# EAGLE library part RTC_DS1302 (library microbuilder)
DS1302 Trickle-Charge Timekeeping Chip
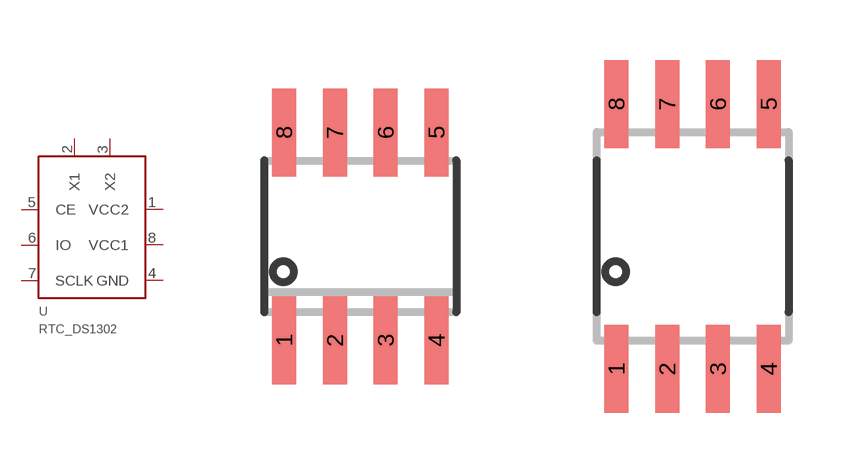
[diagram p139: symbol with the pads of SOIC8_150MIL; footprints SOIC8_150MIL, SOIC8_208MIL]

Designator prefix U

## RTC_DS1302150  [SOIC8_150MIL]
1  VCC2
2  X1
3  X2
4  GND
5  CE
6  IO
7  SCLK
8  VCC1

## RTC_DS1302208  [SOIC8_208MIL]
Pads as for SOIC8_150MIL

## Footprint SOIC8_150MIL (pad centres in mm)
Small Outline IC - 150mil Wide
smd 0.6 x 2.2: 1 -1.905,-2.6; 2 -0.635,-2.6; 3 0.635,-2.6; 4 1.905,-2.6; 5 1.905,2.6; 6 0.635,2.6; 7 -0.635,2.6; 8 -1.905,2.6

## Footprint SOIC8_208MIL (pad centres in mm)
Small Outline IC - 208mil Wide
smd 0.6 x 2.2: 1 -1.905,-3.315; 2 -0.635,-3.315; 3 0.635,-3.315; 4 1.905,-3.315; 5 1.905,3.315; 6 0.635,3.315; 7 -0.635,3.315; 8 -1.905,3.315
